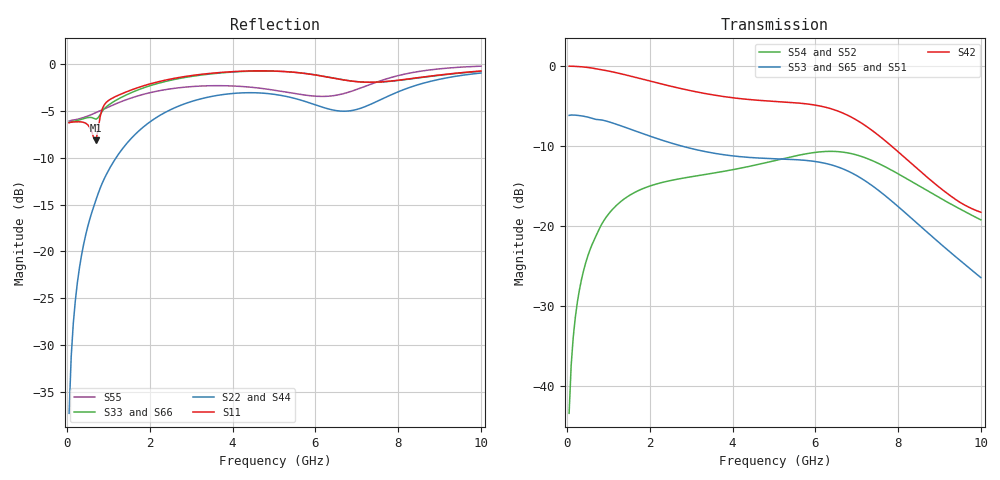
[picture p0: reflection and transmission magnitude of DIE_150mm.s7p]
! Created Wed Jan  2 14:39:17 2019
# ghz S ma R 50
! 7 Port Network Data from SP1.SP block
! freq  magS11  angS11  magS12  angS12  magS13  angS13  magS14  angS14
!  magS15  angS15  magS16  angS16  magS17  angS17
!  magS21  angS21
!  magS22  angS22  magS23  angS23  magS24  angS24  magS25  angS25
!  magS26  angS26  magS27  angS27
!  magS31  angS31  magS32  angS32
!  magS33  angS33  magS34  angS34  magS35  angS35  magS36  angS36
!  magS37  angS37
!  magS41  angS41  magS42  angS42  magS43  angS43
!  magS44  angS44  magS45  angS45  magS46  angS46  magS47  angS47
!  magS51  angS51  magS52  angS52  magS53  angS53  magS54  angS54
!  magS55  angS55  magS56  angS56  magS57  angS57
!  magS61  angS61
!  magS62  angS62  magS63  angS63  magS64  angS64  magS65  angS65
!  magS66  angS66  magS67  angS67
!  magS71  angS71  magS72  angS72
!  magS73  angS73  magS74  angS74  magS75  angS75  magS76  angS76
!  magS77  angS77
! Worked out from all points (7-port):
!   200 points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, 50 MHz to 10 GHz, reference 50 ohm
!   strongest paths, dB at 50 MHz, 2.55 GHz, 5.05 GHz, 7.55 GHz, 10 GHz:
!     S42: 0.0, -2.6, -4.4, -8.8, -18.3
!     S53: -6.2, -9.7, -11.6, -15.7, -26.5
!     S65: -6.2, -9.7, -11.6, -15.7, -26.4
!     S51: -5.9, -9.8, -11.7, -15.7, -26.5
!     S54: -43.5, -14.3, -11.8, -12.2, -19.2
!     S52: -43.5, -14.3, -11.8, -12.2, -19.2
!   lowest |S11| = -8.1 dB at 700 MHz (marker M1), VSWR 2.29, Z = 22.5 - j7.77 ohm
!   |S11| at or under -10 dB: nowhere
